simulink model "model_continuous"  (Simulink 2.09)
settings: Solver=ode1  StartTime=0.0  StopTime=1  FixedStep=0.001  MaxStep=0.001  RelTol=1e-5  AbsTol=1e-5
undefined symbols (not defined in the file or in its folder): movedetect

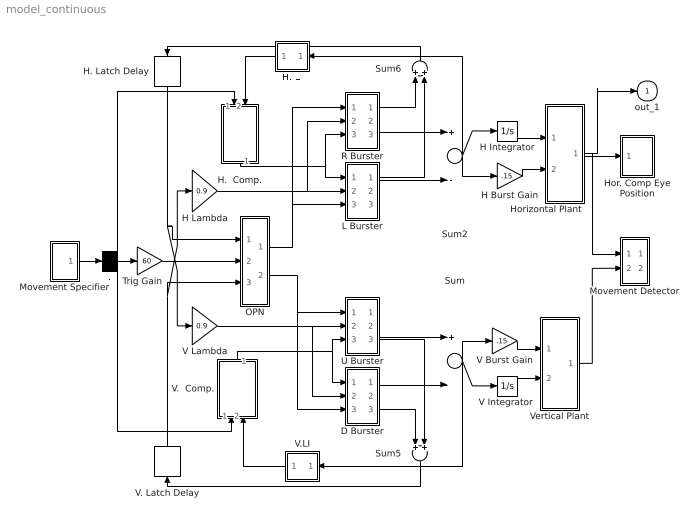
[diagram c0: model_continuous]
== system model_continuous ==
  . : Demux  Outputs=3
  D Burster : Subsystem
  H Burst Gain : Gain  Gain=.15
  H Integrator : Integrator  ExternalReset=none  InitialConditionSource=internal  InitialCondition=0  LimitOutput=off  UpperSaturationLimit=inf  LowerSaturationLimit=-inf  ShowSaturationPort=off  ShowStatePort=off  AbsoluteTolerance=auto
  H Lambda : Gain  Gain=0.9
  H.  Comp. : Subsystem  Orientation=down
  H. LI : Subsystem  Orientation=left
  H. Latch Delay : TransportDelay  Orientation=down  DelayTime=.001  InitialInput=00  BufferSize=1024
  Hor. Comp Eye Position : Subsystem  mask(Graph scope.){}
      mask help: Graph scope using MATLAB graph window. Enter plotting ranges and line type.
      mask init:
      | color = @4; ax = [0, @1, @2, @3]; dt = -1;
  Horizontal Plant : Subsystem
  L Burster : Subsystem
  Movement Detector : Subsystem
  Movement Specifier : Subsystem
  OPN : Subsystem
  R Burster : Subsystem
  Sum : Sum  Inputs=+-
  Sum2 : Sum  Inputs=+-
  Sum5 : Sum  Orientation=down  Inputs=++
  Sum6 : Sum  Orientation=up  Inputs=++
  Trig Gain : Gain  Gain=60
  U Burster : Subsystem
  V Burst Gain : Gain  Gain=.15
  "V Integrator " : Integrator  ExternalReset=none  InitialConditionSource=internal  InitialCondition=0  LimitOutput=off  UpperSaturationLimit=inf  LowerSaturationLimit=-inf  ShowSaturationPort=off  ShowStatePort=off  AbsoluteTolerance=auto
  V Lambda : Gain  Gain=0.9
  V.  Comp. : Subsystem  Orientation=up
  V. Latch Delay : TransportDelay  Orientation=up  DelayTime=.001  InitialInput=00  BufferSize=1024
  V.LI : Subsystem  Orientation=left
  Vertical Plant : Subsystem
  out_1 : Outport  Port=1  InitialOutput=0
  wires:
  ./3 -> V.  Comp./1(in_4)
  Movement Specifier/1(out_1) -> ./1
  ./1 -> H.  Comp./1(in_1)
  ./2 -> Trig Gain/1
  Horizontal Plant/1(out_1) -> out_1/1, Movement Detector/1(Horizontal Position), Hor. Comp Eye Position/1(x)
  Vertical Plant/1(out_1) -> Movement Detector/2(Veritcal Position)
  H Integrator/1 -> Horizontal Plant/1(in_1)
  OPN/2(out_4) -> D Burster/3(in_3), U Burster/1(in_3)
  OPN/1(out_1) -> R Burster/1(in_3), L Burster/3(in_3)
  H. Latch Delay/1 -> V Lambda/1, OPN/1(in_1)
  V. Latch Delay/1 -> H Lambda/1, OPN/3(in_3)
  Trig Gain/1 -> OPN/2(in_2)
  R Burster/1(out_2) -> Sum6/1
  V.LI/1(out_1) -> V.  Comp./2(in_5)
  H. LI/1(out_1) -> H.  Comp./2(in_2)
  Sum5/1 -> V. Latch Delay/1
  Sum6/1 -> H. Latch Delay/1
  L Burster/1(out_1) -> Sum6/2
  V.  Comp./1(out_1) -> D Burster/1(in_1), U Burster/3(in_1)
  V Lambda/1 -> D Burster/2(in_2), U Burster/2(in_2)
  D Burster/2(out_2) -> Sum/2
  D Burster/3(out_3) -> Sum5/1
  U Burster/2(out_3) -> Sum/1
  U Burster/3(out_4) -> Sum5/2
  H Lambda/1 -> R Burster/2(in_2), L Burster/2(in_2)
  R Burster/2(out_3) -> Sum2/1
  L Burster/2(out_2) -> Sum2/2
  H.  Comp./1(out_1) -> R Burster/3(in_1), L Burster/1(in_1)
  Sum/1 -> V.LI/1(in_1), "V Integrator "/1, V Burst Gain/1
  "V Integrator "/1 -> Vertical Plant/2(in_2)
  V Burst Gain/1 -> Vertical Plant/1(in_1)
  Sum2/1 -> H. LI/1(in_1), H Burst Gain/1, H Integrator/1
  H Burst Gain/1 -> Horizontal Plant/2(in_2)

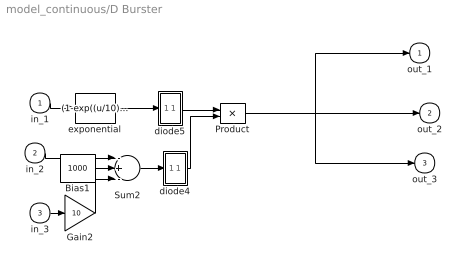
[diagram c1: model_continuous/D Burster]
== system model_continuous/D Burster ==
  in_1 : Inport  Port=1  PortWidth=-1  SampleTime=-1
  in_2 : Inport  Port=2  PortWidth=-1  SampleTime=-1
  in_3 : Inport  Port=3  PortWidth=-1  SampleTime=-1
  Bias1 : Constant  Value=1000
  Gain2 : Gain  Gain=10
  Product : Product  Inputs=2
  Sum2 : Sum  Inputs=-+-
  diode4 : Subsystem
  diode5 : Subsystem
  exponential : Fcn  Expr=(1-exp((u/10)))
  out_1 : Outport  Port=1  InitialOutput=0
  out_2 : Outport  Port=2  InitialOutput=0
  out_3 : Outport  Port=3  InitialOutput=0
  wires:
  in_1/1 -> exponential/1
  Bias1/1 -> Sum2/2
  in_2/1 -> Sum2/1
  in_3/1 -> Gain2/1
  Gain2/1 -> Sum2/3
  Sum2/1 -> diode4/1(in_1)
  diode4/1(out_1) -> Product/2
  exponential/1 -> diode5/1(in_1)
  diode5/1(out_1) -> Product/1
  Product/1 -> out_1/1, out_2/1, out_3/1

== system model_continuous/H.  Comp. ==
  in_1 : Inport  Port=1  PortWidth=-1  SampleTime=-1
  in_2 : Inport  Port=2  PortWidth=-1  SampleTime=-1
  Sum : Sum  Inputs=+-
  out_1 : Outport  Port=1  InitialOutput=0
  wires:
  in_2/1 -> Sum/2
  in_1/1 -> Sum/1
  Sum/1 -> out_1/1

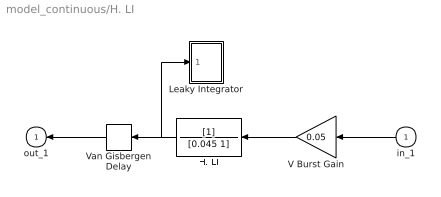
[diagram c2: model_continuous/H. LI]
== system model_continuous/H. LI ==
  in_1 : Inport  Orientation=left  Port=1  PortWidth=-1  SampleTime=-1
  H. LI : TransferFcn  Orientation=left  Numerator=[1]  Denominator=[0.045 1]
  Leaky Integrator : Subsystem  mask(Graph scope.){}
      mask help: Graph scope using MATLAB graph window. Enter plotting ranges and line type.
      mask init:
      | color = @4; ax = [0, @1, @2, @3]; dt = -1;
  V Burst Gain : Gain  Orientation=left  Gain=0.05
  Van Gisbergen Delay : TransportDelay  Orientation=left  DelayTime=.002  InitialInput=00  BufferSize=1024
  out_1 : Outport  Orientation=left  Port=1  InitialOutput=0
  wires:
  Van Gisbergen Delay/1 -> out_1/1
  in_1/1 -> V Burst Gain/1
  V Burst Gain/1 -> H. LI/1
  H. LI/1 -> Van Gisbergen Delay/1, Leaky Integrator/1(x)

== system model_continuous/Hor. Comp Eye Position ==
  x : Inport  Port=1  PortWidth=-1  SampleTime=-1
  "S-function M-file which plots lines " : S-Function  FunctionName=sfuny  Parameters=ax, color,dt
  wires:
  x/1 -> "S-function M-file which plots lines "/1

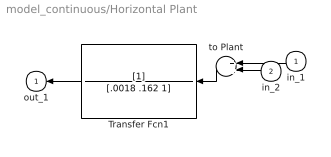
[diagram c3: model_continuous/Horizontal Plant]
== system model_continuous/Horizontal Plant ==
  in_1 : Inport  Orientation=left  Port=1  PortWidth=-1  SampleTime=-1
  in_2 : Inport  Orientation=left  Port=2  PortWidth=-1  SampleTime=-1
  Transfer Fcn1 : TransferFcn  Orientation=left  Numerator=[1]  Denominator=[.0018 .162 1]
  to Plant : Sum  Orientation=left  Inputs=++
  out_1 : Outport  Orientation=left  Port=1  InitialOutput=0
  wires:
  Transfer Fcn1/1 -> out_1/1
  in_2/1 -> to Plant/2
  in_1/1 -> to Plant/1
  to Plant/1 -> Transfer Fcn1/1

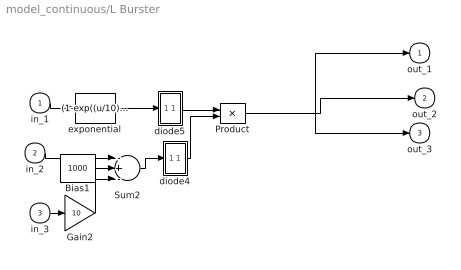
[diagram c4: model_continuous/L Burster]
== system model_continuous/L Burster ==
  in_1 : Inport  Port=1  PortWidth=-1  SampleTime=-1
  in_2 : Inport  Port=2  PortWidth=-1  SampleTime=-1
  in_3 : Inport  Port=3  PortWidth=-1  SampleTime=-1
  Bias1 : Constant  Value=1000
  Gain2 : Gain  Gain=10
  Product : Product  Inputs=2
  Sum2 : Sum  Inputs=-+-
  diode4 : Subsystem
  diode5 : Subsystem
  exponential : Fcn  Expr=(1-exp((u/10)))
  out_1 : Outport  Port=1  InitialOutput=0
  out_2 : Outport  Port=2  InitialOutput=0
  out_3 : Outport  Port=3  InitialOutput=0
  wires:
  Product/1 -> out_3/1, out_2/1, out_1/1
  diode5/1(out_1) -> Product/1
  exponential/1 -> diode5/1(in_1)
  diode4/1(out_1) -> Product/2
  Sum2/1 -> diode4/1(in_1)
  Gain2/1 -> Sum2/3
  in_3/1 -> Gain2/1
  in_2/1 -> Sum2/1
  Bias1/1 -> Sum2/2
  in_1/1 -> exponential/1

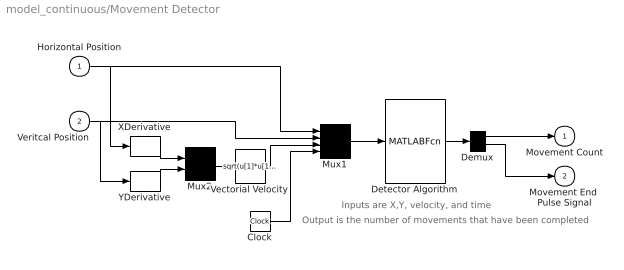
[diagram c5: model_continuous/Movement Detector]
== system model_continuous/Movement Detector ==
  note: Inputs are X,Y, velocity, and time
  note: Output is the number of movements that have been completed
  Horizontal Position : Inport  Port=1  PortWidth=-1  SampleTime=-1
  Veritcal Position : Inport  Port=2  PortWidth=-1  SampleTime=-1
  Clock : Clock
  Demux : Demux  Outputs=2
  Detector Algorithm : MATLABFcn  MATLABFcn=movedetect(u(1),u(2),u(3),u(4))  OutputWidth=2
  Mux1 : Mux  Inputs=4
  Mux2 : Mux  Inputs=2
  Vectorial Velocity : Fcn  Expr=sqrt(u[1]*u[1]+u[2]*u[2])
  XDerivative : Derivative
  YDerivative : Derivative
  Movement Count : Outport  Port=1  InitialOutput=0
  Movement End  Pulse Signal : Outport  Port=2  InitialOutput=0
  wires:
  Demux/2 -> Movement End  Pulse Signal/1
  Demux/1 -> Movement Count/1
  Detector Algorithm/1 -> Demux/1
  Horizontal Position/1 -> XDerivative/1, Mux1/1
  Veritcal Position/1 -> YDerivative/1, Mux1/2
  Vectorial Velocity/1 -> Mux1/3
  Clock/1 -> Mux1/4
  Mux2/1 -> Vectorial Velocity/1
  XDerivative/1 -> Mux2/1
  YDerivative/1 -> Mux2/2
  Mux1/1 -> Detector Algorithm/1

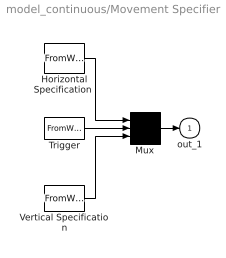
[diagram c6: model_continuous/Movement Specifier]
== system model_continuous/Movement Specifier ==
  "Horizontal Specification " : FromWorkspace  VariableName=hspec
  Mux : Mux  Inputs=3
  Trigger : FromWorkspace  VariableName=trigspec
  Vertical Specification : FromWorkspace  VariableName=vspec
  out_1 : Outport  Port=1  InitialOutput=0
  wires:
  Mux/1 -> out_1/1
  Trigger/1 -> Mux/2
  "Horizontal Specification "/1 -> Mux/1
  Vertical Specification/1 -> Mux/3

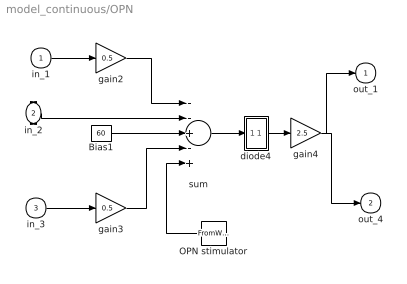
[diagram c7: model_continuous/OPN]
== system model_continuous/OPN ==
  in_1 : Inport  Port=1  PortWidth=-1  SampleTime=-1
  in_2 : Inport  Port=2  PortWidth=-1  SampleTime=-1
  in_3 : Inport  Port=3  PortWidth=-1  SampleTime=-1
  Bias1 : Constant  Value=60
  OPN stimulator : FromWorkspace  Orientation=left  VariableName=stimulate
  diode4 : Subsystem
  gain2 : Gain  Gain=0.5
  gain3 : Gain  Gain=0.5
  gain4 : Gain  Gain=2.5
  sum : Sum  Inputs=--+-+
  out_1 : Outport  Port=1  InitialOutput=0
  out_4 : Outport  Port=2  InitialOutput=0
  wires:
  OPN stimulator/1 -> sum/5
  gain4/1 -> out_4/1, out_1/1
  diode4/1(out_1) -> gain4/1
  gain3/1 -> sum/4
  in_3/1 -> gain3/1
  gain2/1 -> sum/1
  in_1/1 -> gain2/1
  Bias1/1 -> sum/3
  in_2/1 -> sum/2
  sum/1 -> diode4/1(in_1)

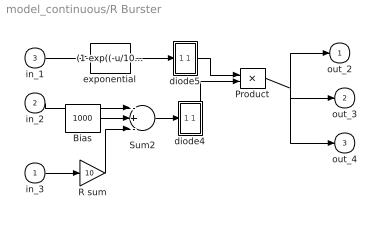
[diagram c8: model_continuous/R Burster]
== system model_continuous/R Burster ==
  in_3 : Inport  Port=1  PortWidth=-1  SampleTime=-1
  in_2 : Inport  Port=2  PortWidth=-1  SampleTime=-1
  in_1 : Inport  Port=3  PortWidth=-1  SampleTime=-1
  Bias : Constant  Value=1000
  Product : Product  Inputs=2
  R sum : Gain  Gain=10
  Sum2 : Sum  Inputs=-+-
  diode4 : Subsystem
  diode5 : Subsystem
  exponential : Fcn  Expr=(1-exp((-u/10)))
  out_2 : Outport  Port=1  InitialOutput=0
  out_3 : Outport  Port=2  InitialOutput=0
  out_4 : Outport  Port=3  InitialOutput=0
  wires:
  diode5/1(out_1) -> Product/1
  exponential/1 -> diode5/1(in_1)
  diode4/1(out_1) -> Product/2
  Sum2/1 -> diode4/1(in_1)
  in_1/1 -> exponential/1
  in_2/1 -> Sum2/1
  Bias/1 -> Sum2/2
  Product/1 -> out_2/1, out_4/1, out_3/1
  in_3/1 -> R sum/1
  R sum/1 -> Sum2/3

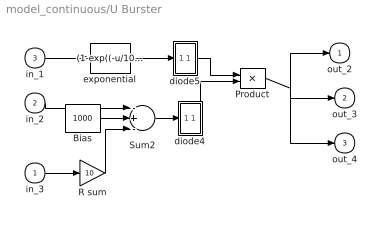
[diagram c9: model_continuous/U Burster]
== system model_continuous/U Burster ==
  in_3 : Inport  Port=1  PortWidth=-1  SampleTime=-1
  in_2 : Inport  Port=2  PortWidth=-1  SampleTime=-1
  in_1 : Inport  Port=3  PortWidth=-1  SampleTime=-1
  Bias : Constant  Value=1000
  Product : Product  Inputs=2
  R sum : Gain  Gain=10
  Sum2 : Sum  Inputs=-+-
  diode4 : Subsystem
  diode5 : Subsystem
  exponential : Fcn  Expr=(1-exp((-u/10)))
  out_2 : Outport  Port=1  InitialOutput=0
  out_3 : Outport  Port=2  InitialOutput=0
  out_4 : Outport  Port=3  InitialOutput=0
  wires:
  diode5/1(out_1) -> Product/1
  exponential/1 -> diode5/1(in_1)
  diode4/1(out_1) -> Product/2
  Sum2/1 -> diode4/1(in_1)
  in_1/1 -> exponential/1
  in_2/1 -> Sum2/1
  Bias/1 -> Sum2/2
  Product/1 -> out_2/1, out_4/1, out_3/1
  in_3/1 -> R sum/1
  R sum/1 -> Sum2/3

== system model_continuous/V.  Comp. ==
  in_4 : Inport  Port=1  PortWidth=-1  SampleTime=-1
  in_5 : Inport  Port=2  PortWidth=-1  SampleTime=-1
  Sum : Sum  Inputs=-+
  out_1 : Outport  Port=1  InitialOutput=0
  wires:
  in_4/1 -> Sum/2
  in_5/1 -> Sum/1
  Sum/1 -> out_1/1

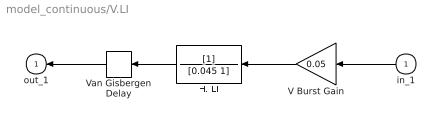
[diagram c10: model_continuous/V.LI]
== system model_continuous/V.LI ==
  in_1 : Inport  Orientation=left  Port=1  PortWidth=-1  SampleTime=-1
  H. LI : TransferFcn  Orientation=left  Numerator=[1]  Denominator=[0.045 1]
  V Burst Gain : Gain  Orientation=left  Gain=0.05
  Van Gisbergen Delay : TransportDelay  Orientation=left  DelayTime=.002  InitialInput=00  BufferSize=1024
  out_1 : Outport  Orientation=left  Port=1  InitialOutput=0
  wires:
  H. LI/1 -> Van Gisbergen Delay/1
  V Burst Gain/1 -> H. LI/1
  in_1/1 -> V Burst Gain/1
  Van Gisbergen Delay/1 -> out_1/1

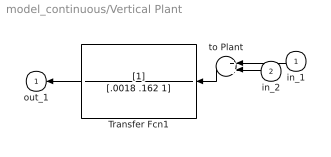
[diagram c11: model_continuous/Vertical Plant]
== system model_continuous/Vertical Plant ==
  in_1 : Inport  Orientation=left  Port=1  PortWidth=-1  SampleTime=-1
  in_2 : Inport  Orientation=left  Port=2  PortWidth=-1  SampleTime=-1
  Transfer Fcn1 : TransferFcn  Orientation=left  Numerator=[1]  Denominator=[.0018 .162 1]
  to Plant : Sum  Orientation=left  Inputs=++
  out_1 : Outport  Orientation=left  Port=1  InitialOutput=0
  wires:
  Transfer Fcn1/1 -> out_1/1
  in_2/1 -> to Plant/2
  in_1/1 -> to Plant/1
  to Plant/1 -> Transfer Fcn1/1

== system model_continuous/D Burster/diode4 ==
  in_1 : Inport  Port=1  PortWidth=-1  SampleTime=-1
  Switch : Switch  Threshold=0
  diode1 : Constant  Value=0
  out_1 : Outport  Port=1  InitialOutput=0
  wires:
  in_1/1 -> Switch/2, Switch/1
  Switch/1 -> out_1/1
  diode1/1 -> Switch/3

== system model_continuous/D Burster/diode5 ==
  in_1 : Inport  Port=1  PortWidth=-1  SampleTime=-1
  Switch : Switch  Threshold=0
  diode1 : Constant  Value=0
  out_1 : Outport  Port=1  InitialOutput=0
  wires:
  in_1/1 -> Switch/2, Switch/1
  Switch/1 -> out_1/1
  diode1/1 -> Switch/3

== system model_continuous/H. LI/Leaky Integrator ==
  x : Inport  Port=1  PortWidth=-1  SampleTime=-1
  "S-function M-file which plots lines " : S-Function  FunctionName=sfuny  Parameters=ax, color,dt
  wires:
  x/1 -> "S-function M-file which plots lines "/1

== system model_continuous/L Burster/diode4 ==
  in_1 : Inport  Port=1  PortWidth=-1  SampleTime=-1
  Switch : Switch  Threshold=0
  diode1 : Constant  Value=0
  out_1 : Outport  Port=1  InitialOutput=0
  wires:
  diode1/1 -> Switch/3
  Switch/1 -> out_1/1
  in_1/1 -> Switch/2, Switch/1

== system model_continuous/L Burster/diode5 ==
  in_1 : Inport  Port=1  PortWidth=-1  SampleTime=-1
  Switch : Switch  Threshold=0
  diode1 : Constant  Value=0
  out_1 : Outport  Port=1  InitialOutput=0
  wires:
  diode1/1 -> Switch/3
  Switch/1 -> out_1/1
  in_1/1 -> Switch/2, Switch/1

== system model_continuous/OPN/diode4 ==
  in_1 : Inport  Port=1  PortWidth=-1  SampleTime=-1
  Switch : Switch  Threshold=0
  diode1 : Constant  Value=0
  out_1 : Outport  Port=1  InitialOutput=0
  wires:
  in_1/1 -> Switch/2, Switch/1
  Switch/1 -> out_1/1
  diode1/1 -> Switch/3

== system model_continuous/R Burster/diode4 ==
  in_1 : Inport  Port=1  PortWidth=-1  SampleTime=-1
  Switch : Switch  Threshold=0
  diode1 : Constant  Value=0
  out_1 : Outport  Port=1  InitialOutput=0
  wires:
  in_1/1 -> Switch/2, Switch/1
  Switch/1 -> out_1/1
  diode1/1 -> Switch/3

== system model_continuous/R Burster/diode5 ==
  in_1 : Inport  Port=1  PortWidth=-1  SampleTime=-1
  Switch : Switch  Threshold=0
  diode1 : Constant  Value=0
  out_1 : Outport  Port=1  InitialOutput=0
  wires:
  diode1/1 -> Switch/3
  Switch/1 -> out_1/1
  in_1/1 -> Switch/2, Switch/1

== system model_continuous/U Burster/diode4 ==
  in_1 : Inport  Port=1  PortWidth=-1  SampleTime=-1
  Switch : Switch  Threshold=0
  diode1 : Constant  Value=0
  out_1 : Outport  Port=1  InitialOutput=0
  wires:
  in_1/1 -> Switch/2, Switch/1
  Switch/1 -> out_1/1
  diode1/1 -> Switch/3

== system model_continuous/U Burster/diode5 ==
  in_1 : Inport  Port=1  PortWidth=-1  SampleTime=-1
  Switch : Switch  Threshold=0
  diode1 : Constant  Value=0
  out_1 : Outport  Port=1  InitialOutput=0
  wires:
  diode1/1 -> Switch/3
  Switch/1 -> out_1/1
  in_1/1 -> Switch/2, Switch/1
